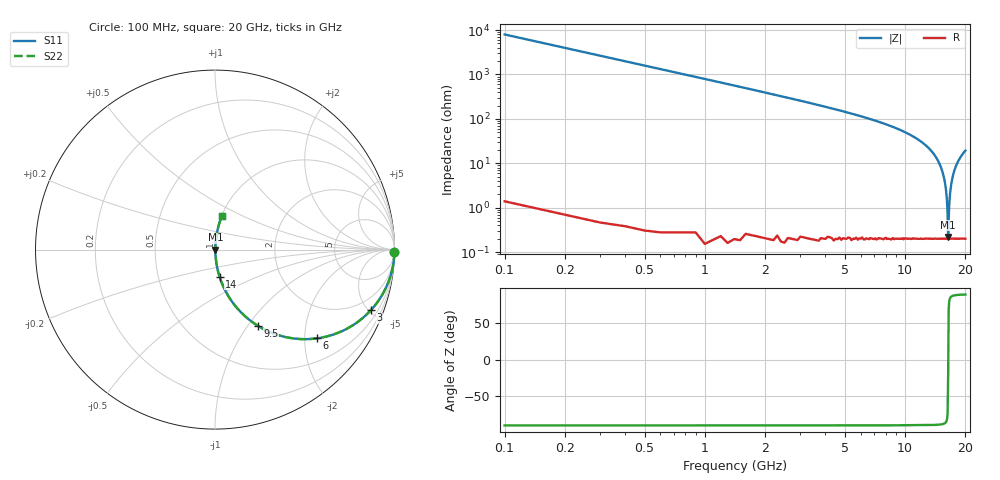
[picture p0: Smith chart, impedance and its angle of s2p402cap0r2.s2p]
! AVX Thin Film Operation		Date: April 2003
! Description: Accu-P® Series, Thin Film, SMD, RF Capacitor
! Part Number: 04023J0R2ABW
! 50 MHz  -  20 GHz
! Serial Measurements
# hz S db R 50
!	S11		S21		S12		S22
!	dB	Phase	dB	Phase	dB	Phase	dB	Phase
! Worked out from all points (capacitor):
!   200 points, 100 MHz to 20 GHz, reference 50 ohm
!   read as one part in series: C = 200 fF near 200 MHz
!   lowest |Z| = 220 mohm at 16.4 GHz (marker M1)
!   series resonance near 16.42 GHz, so ESL is about 470 pH
!   S11 on the Smith chart (normalised r, x): 100 MHz: open; 3 GHz: 1.00, -5.13; 6 GHz: 1.00, -2.30; 9.5 GHz: 1.00, -1.11; 14 GHz: 1.00, -0.31; 20 GHz: 1.00, +0.39
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1e8  -0.00 -0.7  -38.02 89.3  -38.02 89.3  -0.00 -0.7
2e8  -0.00 -1.4  -32.00 88.5  -32.00 88.5  -0.00 -1.4
4e8  -0.01 -2.9  -25.98 87.1  -25.98 87.1  -0.01 -2.9
9e8  -0.06 -6.5  -18.96 83.5  -18.96 83.5  -0.06 -6.5
3e9  -0.62 -21.3  -8.80 68.7  -8.80 68.7  -0.62 -21.3
3.5e9  -0.84 -24.7  -7.57 65.2  -7.57 65.2  -0.84 -24.7
6e9  -2.46 -41.0  -3.66 48.9  -3.66 48.9  -2.46 -41.0
6.8e9  -3.16 -45.8  -2.89 44.0  -2.89 44.0  -3.16 -45.8
9.5e9  -6.27 -60.7  -1.19 29.1  -1.19 29.1  -6.27 -60.7
1.01e10  -7.15 -63.7  -0.95 26.0  -0.95 26.0  -7.15 -63.7
1.34e10  -14.24 -78.2  -0.18 11.2  -0.18 11.2  -14.24 -78.2
1.4e10  -16.31 -80.5  -0.12 8.8  -0.12 8.8  -16.31 -80.5
1.51e10  -21.86 -84.0  -0.05 4.6  -0.05 4.6  -21.86 -84.0
1.58e10  -28.63 -84.8  -0.02 2.1  -0.02 2.1  -28.63 -84.8
1.62e10  -37.76 -80.4  -0.02 0.7  -0.02 0.7  -37.76 -80.4
1.63e10  -42.95 -73.3  -0.02 0.4  -0.02 0.4  -42.95 -73.3
1.64e10  -53.16 -24.7  -0.02 0.1  -0.02 0.1  -53.16 -24.7
1.66e10  -39.18 78.9  -0.02 -0.6  -0.02 -0.6  -39.18 78.9
1.67e10  -35.53 82.2  -0.02 -1.0  -0.02 -1.0  -35.53 82.2
1.71e10  -28.06 84.8  -0.02 -2.3  -0.02 -2.3  -28.06 84.8
1.77e10  -22.76 84.3  -0.04 -4.2  -0.04 -4.2  -22.76 84.3
2e10  -14.48 78.5  -0.18 -10.9  -0.18 -10.9  -14.48 78.5
